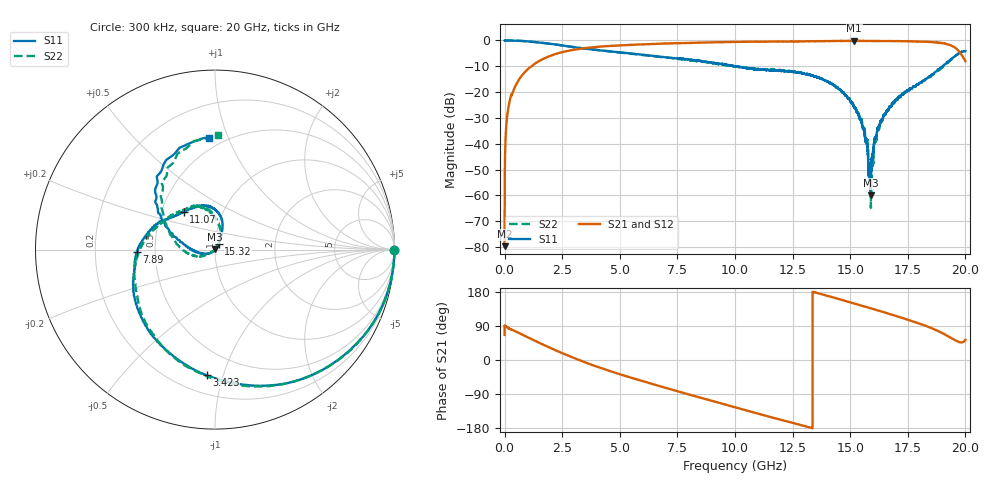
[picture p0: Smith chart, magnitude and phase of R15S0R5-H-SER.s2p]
!{R15S0R5}
!Johanson Technology Inc.
!www.johansontechnology.com
!Test Board Conditions:
!Substrate Type  RO4350B
!Substrate Thickness  20 mil
!Substrate Dk  3.66
!TL Type: GCPW
!TL Trace Width  34 mil
!TL Gap  10 mil
!Electrode orientation  Horizontal
!DUT TOPOLOGY	SERIES
!Mounting Pad LxW  26x52 mil
! Created Sat Feb  6 12:06:14 2021
# hz S ma R 50
! 2 Port Network Data from SP1.SP block
! freq  magS11  angS11  magS21  angS21  magS12  angS12  magS22  angS22
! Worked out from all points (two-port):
!   20001 points, 300 kHz to 20 GHz, reference 50 ohm
!   highest |S21| = -0.14 dB at 15.18 GHz (marker M1); lowest = -79.6 dB at 300 kHz (marker M2)
!   |S21| within 3 dB of the highest: 3.351 GHz to 19.61 GHz (16.25 GHz wide, 142 % of centre)
!   lowest |S11| = -59.9 dB at 15.89 GHz (marker M3), VSWR 1.00, Z = 49.9 + j0.0629 ohm
!   |S11| at or under -10 dB: 10.01491 GHz to 10.01601 GHz (1.092 MHz wide, 0.0109 % of centre); 10.01649 GHz to 10.01773 GHz (1.241 MHz wide, 0.0124 % of centre); 10.02 GHz to 19.01 GHz (8.99 GHz wide, 61.9 % of centre)
!   |S22| runs from -64.8 to 0.0 dB; largest |S21 - S12| = 0.013
!   S11 on the Smith chart (normalised r, x): 300 kHz: open; 3.423 GHz: 0.32, -0.88; 7.89 GHz: 0.39, -0.01; 11.07 GHz: 0.65, +0.29; 15.32 GHz: 1.04, +0.07; 20 GHz: 0.43, +0.86
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300000  0.9947 -0.0  0.0001043 66.2  0.0001127 68.1  0.9954 -0.2
1.013e8  0.9995 -3.3  0.03116 86.5  0.03138 86.4  0.9988 -3.3
1.363e8  0.9979 -4.4  0.04186 85.2  0.0421 85.3  0.999 -4.4
5.183e8  0.9889 -15.3  0.1455 74.4  0.1459 74.4  0.9884 -15.5
1.8613e9  0.8761 -54.3  0.4782 35.3  0.4792 35.3  0.8733 -54.8
3.3343e9  0.7104 -91.8  0.6953 -2.5  0.6968 -2.5  0.7104 -92.7
3.4233e9  0.7015 -93.8  0.703 -4.6  0.7046 -4.6  0.7026 -94.9
6.6673e9  0.4896 -158.5  0.8613 -67.9  0.8631 -67.8  0.4819 -157.2
7.8903e9  0.4351 -178.4  0.8935 -89.0  0.8973 -89.0  0.4229 -179.0
1.00003e10  0.3194 147.6  0.9375 -124.8  0.9407 -124.8  0.3153 144.7
1.10723e10  0.2725 129.9  0.9484 -142.6  0.9504 -142.9  0.2761 125.3
1.33343e10  0.2081 85.1  0.9654 -179.5  0.9626 -179.5  0.2081 96.9
1.51773e10  0.05086 60.0  0.9843 149.0  0.9779 149.0  0.05076 60.8
1.53193e10  0.03945 58.3  0.9783 146.5  0.9754 146.6  0.03989 56.7
1.56683e10  0.01187 47.5  0.9768 140.5  0.98 140.6  0.01203 55.4
1.58103e10  0.002482 44.0  0.9763 137.9  0.9788 137.9  0.002949 53.9
1.58853e10  0.001012 141.5  0.977 136.5  0.9768 136.7  0.002415 50.3
1.61363e10  0.01436 -140.3  0.9782 132.0  0.9751 132.1  0.01205 -141.7
1.66673e10  0.04618 -152.3  0.9769 122.2  0.9691 122.3  0.04757 -147.6
1.87713e10  0.2606 159.2  0.9099 77.6  0.913 77.7  0.2491 163.4
1.95383e10  0.4886 130.9  0.7311 52.8  0.73 53.5  0.4864 125.0
2e10  0.6201 92.5  0.3968 53.5  0.391 53.8  0.6364 88.2
